(* Logix 5000 AddOnInstructionDefinition export AMCI_SV160E2_Enable; software revision 20.03 *)

ADD_ON_INSTRUCTION AMCI_SV160E2_Enable   (* revision 1.0, vendor AMCI *)
// Revision note:
// 8/2019 Version 0 Initial release of SV160E2 Add On Instructions.
// 3/17/20 Version 1 replaced the generic EDS file with a more complete V1.6 EDS file.
VAR_IN_OUT
   AMCI_SV160E2_OUTPUT_DATA : _000A:SV160E2_9125ACD4:O:0; {required}
END_VAR
VAR
   command_data_block : INT[10];
        [0]   // Command Bits MSW
        [1]   // Command Bits LSW
        [2]   // Upper Target Position
        [3]   // Lower Target Position
        [4]   // Upper Programmed Speed
        [5]   // Lower Programmed Speed
END_VAR

ROUTINE Logic   (* ladder *)
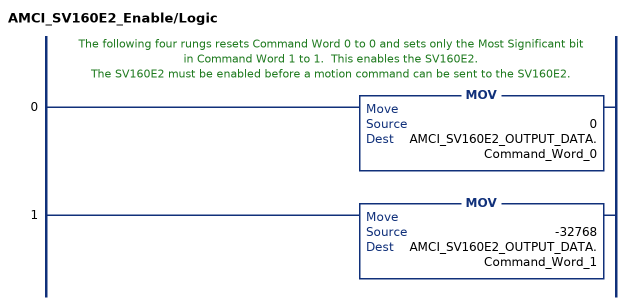
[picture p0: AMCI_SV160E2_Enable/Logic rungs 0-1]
   // The following four rungs resets Command Word 0 to 0 and sets only the Most Significant bit in Command Word 1 to 1.  This enables the SV160E2.
   // The SV160E2 must be enabled before a motion command can be sent to the SV160E2.
   0: MOV(0,AMCI_SV160E2_OUTPUT_DATA.Command_Word_0);
   1: MOV(-32768,AMCI_SV160E2_OUTPUT_DATA.Command_Word_1);
END_ROUTINE
END_ADD_ON_INSTRUCTION
